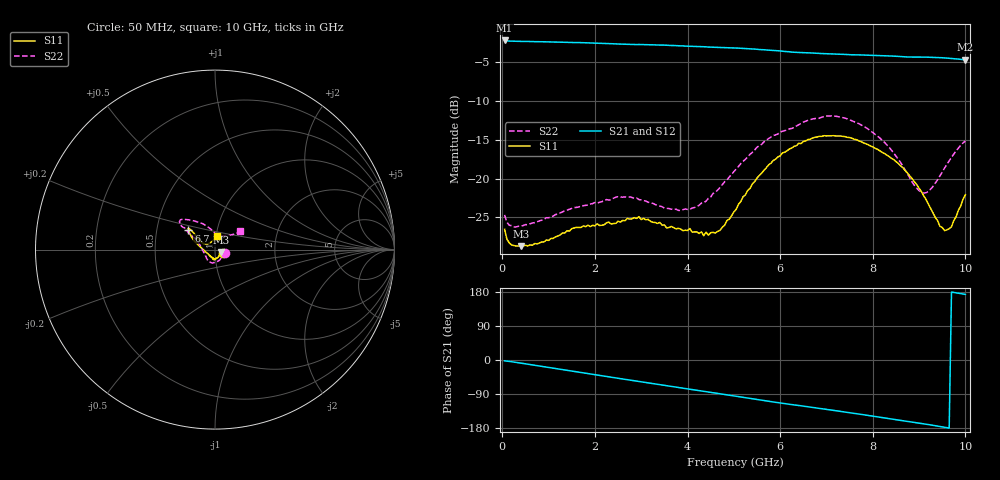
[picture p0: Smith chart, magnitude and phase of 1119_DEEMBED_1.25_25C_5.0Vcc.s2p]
!Hittite Microwave Corp.
!Digital Attenuator/PhaseShifter Rev 1.4.0
!Filename: C:\DATA\DATA\1119_DEEMBED_1.25_25C_5.0Vcc.s2p
!VNA ID: Agilent Technologies,N5224A,MY51441122,A.10.45.03
!Device type:
!2 Port Calibration.
!Temp(C): 25
!Lot Number:
!Serial Number:
!Operator:
!Misc:
!Attenuator:  1.250
# GHZ S DB R 50.0
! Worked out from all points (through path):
!   200 points, 50 MHz to 10 GHz, reference 50 ohm
!   highest |S21| = -2.18 dB at 50 MHz (marker M1); lowest = -4.7 dB at 10 GHz (marker M2)
!   group delay of S21, straight-line fit = 51.1 ps
!   lowest |S11| = -28.7 dB at 400 MHz (marker M3), VSWR 1.08, Z = 53.4 - j1.6 ohm
!   |S11| at or under -10 dB: start of sweep to end of sweep
!   |S22| runs from -26.2 to -11.9 dB; largest |S21 - S12| = 0.0028
!   S11 on the Smith chart (normalised r, x): 50 MHz: 1.09, -0.04; 6.7 GHz: 0.73, +0.16; 10 GHz: 1.01, +0.16
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0.05  -26.53 -24.8  -2.18 -2.3  -2.17 -2.3  -24.68 -18.5
0.15  -28.28 -18.8  -2.26 -3.6  -2.25 -3.6  -26.01 -15.8
0.4  -28.71 -24.0  -2.30 -8.2  -2.30 -8.2  -26.12 -22.7
1.75  -26.09 -80.1  -2.47 -34.0  -2.47 -34.1  -23.49 -76.3
2.5  -25.49 -89.1  -2.64 -48.3  -2.65 -48.4  -22.33 -101.8
2.95  -24.91 -96.0  -2.70 -56.4  -2.71 -56.5  -22.70 -120.3
3.4  -25.65 -103.2  -2.77 -64.9  -2.77 -65.0  -23.51 -135.7
4.05  -26.43 -113.5  -2.92 -77.1  -2.92 -77.1  -23.98 -162.9
4.45  -27.29 -134.6  -3.03 -84.5  -3.04 -84.6  -22.54 175.3
4.7  -26.68 -152.9  -3.08 -89.1  -3.10 -89.2  -21.15 163.1
5.05  -23.97 -178.2  -3.16 -95.7  -3.17 -95.7  -18.77 152.9
5.85  -17.66 156.0  -3.47 -110.7  -3.49 -110.8  -14.44 145.9
6.7  -14.77 144.2  -3.80 -125.2  -3.81 -125.3  -12.31 143.1
7.4  -14.58 141.1  -3.98 -137.3  -4.00 -137.4  -12.19 136.3
7.9  -15.62 141.2  -4.07 -146.3  -4.08 -146.3  -13.61 128.6
8.35  -17.14 143.1  -4.17 -154.6  -4.18 -154.7  -15.94 115.4
8.9  -20.41 149.8  -4.32 -164.5  -4.33 -164.5  -20.87 90.0
9.1  -22.22 151.3  -4.33 -168.3  -4.36 -168.3  -21.86 75.9
9.3  -24.42 148.4  -4.36 -172.3  -4.38 -172.3  -21.02 59.4
9.55  -26.70 127.0  -4.43 -177.5  -4.46 -177.5  -18.63 43.7
9.7  -26.20 106.2  -4.51 179.3  -4.53 179.4  -17.25 38.9
10  -22.08 80.8  -4.67 173.1  -4.69 173.2  -15.15 35.8
